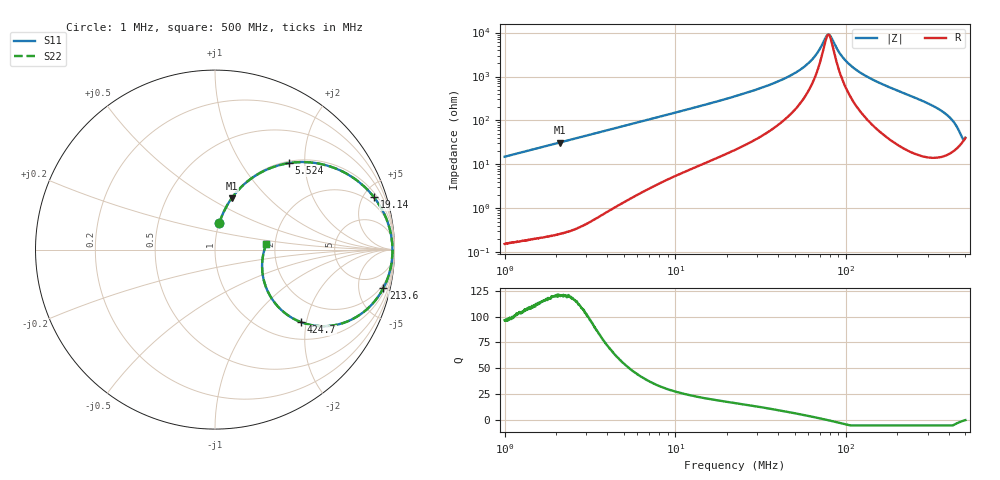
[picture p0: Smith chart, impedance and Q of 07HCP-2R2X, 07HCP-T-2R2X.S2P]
!s-Parameter Generated by FASTRON Sdn. Bhd.
!FASTRON P/N : 07HCP-2R2X, 07HCP/T-2R2X
!Keysight Technologies,E4991B,MY54100416,A.01.15
!Date: Thu Feb 19 16:07:07 2026
!Version  : Rev00 Thu Feb 19 16:07:07 2026
!Data & Calibration Information:
!PortZ  Port1:50+j0  Port2:50+j0
!When reading, reference impedance value at option line is always used.
! Remarks : This data is being provided solely for informational purposes.
!Freq	S11	S21	S12	S22
# Hz S dB R 50
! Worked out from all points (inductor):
!   1601 points, 1 MHz to 500 MHz, reference 50 ohm
!   read as one part in series: L = 2.38 uH near 1.032 MHz
!   highest Q = 120 at 2.108 MHz (marker M1), where L = 2.38 uH
!   self-resonance near 78.84 MHz
!   S11 on the Smith chart (normalised r, x): 1 MHz: 1.00, +0.30; 5.524 MHz: 1.03, +1.66; 19.14 MHz: 1.33, +5.94; 213.6 MHz: 1.48, -8.62; 424.7 MHz: 1.40, -1.86; 500 MHz: 1.80, +0.13
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1000000  -16.62 80.9  -0.11 -8.5  -0.11 -8.5  -16.62 80.9
2108028  -10.47 72.1  -0.43 -17.4  -0.43 -17.4  -10.47 72.1
2820919  -8.23 66.7  -0.74 -22.8  -0.74 -22.8  -8.23 66.7
5523530  -3.98 49.6  -2.37 -39.2  -2.37 -39.2  -3.98 49.6
7957584  -2.42 39.1  -3.99 -49.1  -3.99 -49.1  -2.42 39.1
1.914303e7  -0.61 18.2  -10.08 -68.6  -10.08 -68.6  -0.61 18.2
2.236068e7  -0.47 15.5  -11.46 -71.1  -11.46 -71.1  -0.47 15.5
4.344476e7  -0.16 6.3  -19.18 -77.1  -19.18 -77.1  -0.16 6.3
5.379161e7  -0.12 3.9  -23.18 -76.2  -23.18 -76.2  -0.12 3.9
6.307767e7  -0.11 2.3  -27.73 -71.6  -27.73 -71.6  -0.11 2.3
7.659818e7  -0.10 0.3  -38.34 -24.7  -38.34 -24.7  -0.10 0.3
7.932318e7  -0.10 -0.1  -39.21 5.7  -39.21 5.7  -0.10 -0.1
9.337876e7  -0.10 -1.7  -29.86 68.8  -29.86 68.8  -0.10 -1.7
1.069764e8  -0.11 -3.2  -24.96 76.0  -24.96 76.0  -0.11 -3.2
1.319406e8  -0.13 -5.6  -20.18 78.2  -20.18 78.2  -0.13 -5.6
1.77937e8  -0.22 -9.7  -15.45 76.5  -15.45 76.5  -0.22 -9.7
2.135741e8  -0.33 -12.9  -13.03 73.9  -13.03 73.9  -0.33 -12.9
3.299715e8  -1.15 -25.2  -7.40 60.9  -7.40 60.9  -1.15 -25.2
3.780214e8  -2.06 -32.2  -5.41 51.7  -5.41 51.7  -2.06 -32.2
4.247389e8  -4.06 -40.2  -3.61 37.8  -3.61 37.8  -4.06 -40.2
4.680513e8  -8.78 -37.5  -2.56 17.3  -2.56 17.3  -8.78 -37.5
5e8  -10.80 6.4  -2.92 -2.6  -2.92 -2.6  -10.80 6.4
